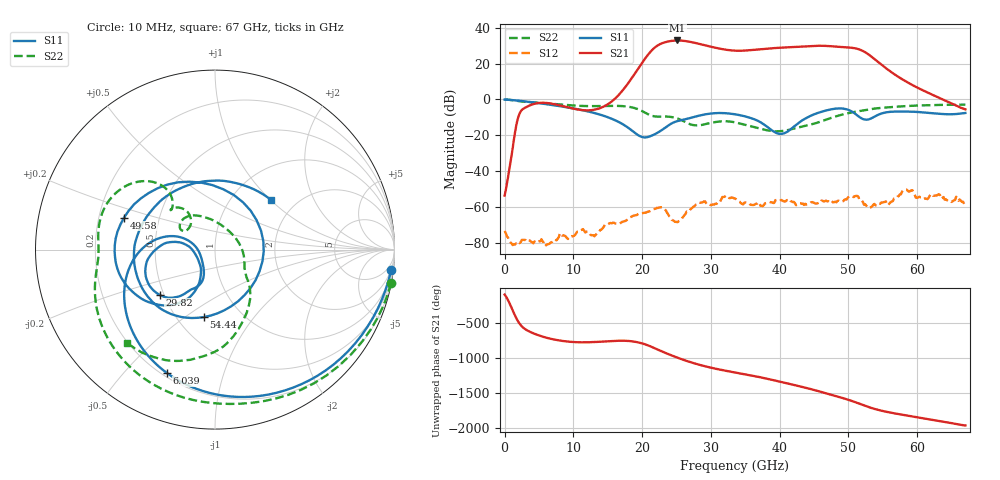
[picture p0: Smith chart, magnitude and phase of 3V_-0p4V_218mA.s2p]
! MARKI MICROWAVE INC.
! Date:  10/23/18
! Model Number:  AMM-6702CH
! Description:  2-port Small Signal S-parameter data for AMM-6702CH
! Frequency Range:  10 MHz to 67 GHz
! Port Configuration:  PORT 1: Input
!  PORT 2: Output
! Bias Condition: Vd = +3V, Vg = -0.4V
! AMM-6702CH s2p files are only valid for small signal conditions (below -5 dBm input power)
!S2P File: Measurements: Mag<S11> Ang<S11>, Mag<S21> Ang<S21>, Mag<S12> Ang<S12>, Mag<S22> Ang<S22>!row 1
# Hz S  dB  R 50
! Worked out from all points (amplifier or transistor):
!   401 points, 10 MHz to 67 GHz, reference 50 ohm
!   highest |S21| = 32.9 dB at 25.13 GHz (marker M1)
!   |S21| within 3 dB of that: 22.18 GHz to 29.47 GHz (7.29 GHz wide, 28.2 % of centre)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
!   unconditionally stable (mu >= 1): start of sweep to end of sweep
!   at 11.06 GHz: K = 1838.74, MAG = -2.1 dB, |S12| = -73.0 dB
!   at 33.51 GHz: K = 10.21, MAG = 28.1 dB, |S12| = -55.3 dB
!   at 67 GHz: K = 353.30, MAG = -1.6 dB, |S12| = -59.3 dB
!   S11 on the Smith chart (normalised r, x): 10 MHz: 2, -17; 6.039 GHz: 0.22, -0.66; 29.82 GHz: 0.47, -0.28; 49.58 GHz: 0.31, +0.15; 54.44 GHz: 0.67, -0.59; 67 GHz: 1.50, +1.01
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1e7  -0.11 -6.7  -53.68 -94.8  -73.36 18.3  -0.02 -10.8
6.0391e9  -2.65 -111.4  -1.98 11.4  -81.33 70.4  -2.17 -138.9
1.123082e10  -5.96 -165.3  -5.95 -55.5  -72.76 155.8  -3.66 -174.0
1.993952e10  -20.93 -171.7  20.07 -69.1  -63.53 138.8  -6.42 130.3
2.14468e10  -20.14 -135.6  27.51 -122.6  -61.58 124.3  -9.19 132.7
2.245165e10  -18.13 -120.6  30.51 -166.6  -60.34 102.8  -9.64 137.9
2.362398e10  -15.10 -112.2  32.16 144.0  -63.17 59.9  -9.60 136.4
2.513125e10  -12.12 -118.8  32.87 86.3  -68.51 110.4  -10.64 128.6
2.714095e10  -10.22 -125.4  31.97 18.6  -60.96 137.2  -14.06 132.7
2.982055e10  -7.98 -140.8  29.54 -52.4  -58.66 107.4  -13.26 149.9
3.3505e10  -8.30 -170.4  27.18 -124.4  -55.28 39.1  -12.79 124.0
3.735692e10  -13.07 168.9  28.03 163.1  -59.41 51.9  -16.47 84.6
4.053895e10  -19.02 -143.4  28.91 92.9  -56.79 7.0  -17.57 26.8
4.254865e10  -13.76 -115.5  29.29 46.5  -58.71 -135.9  -15.85 -9.8
4.472582e10  -8.77 -124.6  29.82 -6.9  -57.29 39.5  -13.88 -34.9
4.723795e10  -5.75 -153.0  29.70 -75.5  -57.37 -133.7  -10.63 -48.6
4.95826e10  -5.40 160.7  29.06 -141.9  -55.68 77.6  -8.01 -64.1
5.09224e10  -7.86 110.7  28.53 174.6  -54.00 162.7  -6.98 -71.7
5.209472e10  -10.94 35.1  27.01 131.9  -57.21 -30.3  -6.14 -77.9
5.443938e10  -8.39 -99.2  20.44 59.1  -57.96 -57.0  -4.84 -90.8
5.594665e10  -6.99 -132.7  15.98 26.5  -58.13 73.2  -4.38 -97.7
6.7e10  -7.58 41.6  -5.54 -159.7  -59.30 32.0  -2.93 -133.3
